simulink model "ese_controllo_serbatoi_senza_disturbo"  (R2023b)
settings: Solver=ode45  StartTime=0.0  StopTime=50  RelTol=1e-3  EnableMultiTasking=on
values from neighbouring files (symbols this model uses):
  k = [0:0.1:8]    [ese_controllo_serbatoi.m]

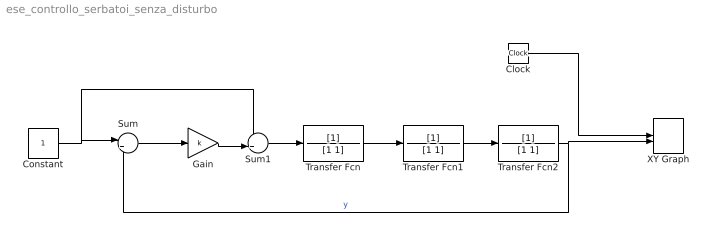
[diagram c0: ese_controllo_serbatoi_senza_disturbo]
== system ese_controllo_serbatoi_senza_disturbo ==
  Clock : Clock
  Constant : Constant
  Gain : Gain  Gain=k
  Sum : Sum  Inputs=|+-
  Sum1 : Sum  Inputs=++|
  Transfer Fcn : TransferFcn  Denominator=[1 1]
  Transfer Fcn1 : TransferFcn  Denominator=[1 1]
  Transfer Fcn2 : TransferFcn  Denominator=[1 1]
  XY Graph : Record  FileSettingsInternal="{\"entries\":[{\"content\":{\"excelSettings\":{\"content\":{},\"type\":\"Streamout.ExcelSettings\"}},\"type\":\"Streamout.FileSettingStorage\",\"uuid\":\"\"}],\"packageUris\":[\"http:\\/\\/schema.mathworks.com\\/mf0\\/streamout_blocks\\/R2020a\"],\"version\":\"1.0\"}"  Layout=[1 1]  SignalsInternal="{\"entries\":[{\"content\":{\"signals\":[{\"content\":{\"blockPath\":[],\"dimensions\":[1],\"domain\":\"\",\"lineColor\":\"#a2142f\",\"plots\":[ 1 ],\"port\":1,\"sid\":[\"\"],\"signalID\":1,\"signalName\":\"Clock\"},\"type\":\"RecordBlkView.Signal\",\"uuid\":\"\"},{\"content\":{\"blockPath\":[],\"dimensions\":[1],\"domain\":\"\",\"lineColor\":\"#139fff\",\"plots\":[ 1 ],\"port\":2,\"sid\":[\"\"],\"signalID\":2,\"signalName\":\"y\"},\"type\":\"RecordBlkView.Signal\",\"uui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"  VisualizationBindings="{\"xyplotplugin\":{\"info\":[{\"series\":[{\"bindingParametersList\":[{\"parameter\":\"X-Axis\",\"signalID\":1,\"signalName\":\"Clock\"},{\"parameter\":\"Y-Axis\",\"signalID\":2,\"signalName\":\"y\"}],\"seriesID\":0}],\"subplotID\":1}]}}"  CompatibilityTag=XY  st=0.01
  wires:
  Transfer Fcn/1 -> Transfer Fcn1/1
  Transfer Fcn1/1 -> Transfer Fcn2/1
  Transfer Fcn2/1 -> Sum/2, XY Graph/2  "y"
  Clock/1 -> XY Graph/1
  Constant/1 -> Sum/1, Sum1/1
  Sum/1 -> Gain/1
  Gain/1 -> Sum1/2
  Sum1/1 -> Transfer Fcn/1
